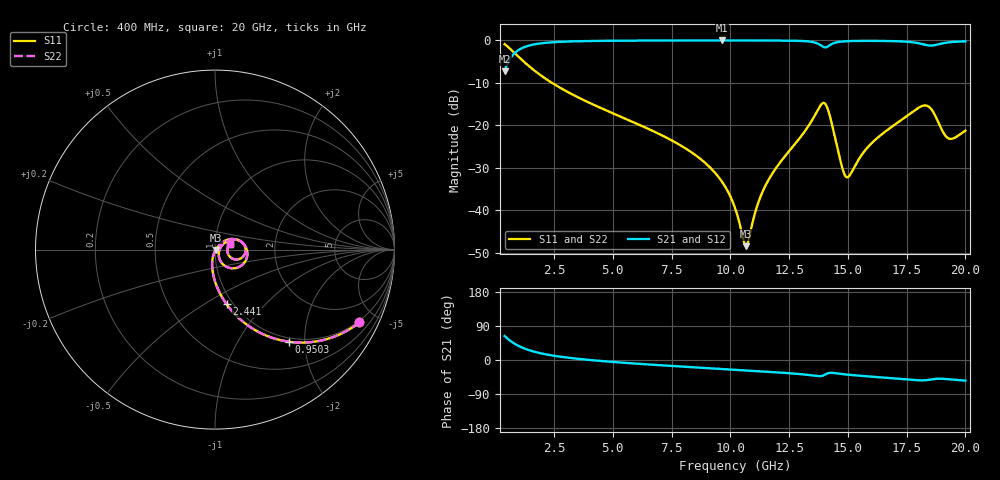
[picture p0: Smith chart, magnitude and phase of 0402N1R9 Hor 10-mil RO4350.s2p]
# GHz S MA R 50
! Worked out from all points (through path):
!   1960 points, 400 MHz to 20 GHz, reference 50 ohm
!   highest |S21| = -0.03 dB at 9.635 GHz (marker M1); lowest = -7.3 dB at 400 MHz (marker M2)
!   group delay of S21, straight-line fit = 11.7 ps
!   lowest |S11| = -48.5 dB at 10.67 GHz (marker M3), VSWR 1.01, Z = 50.3 - j0.195 ohm
!   |S11| at or under -10 dB: 2.407 GHz to end of sweep
!   |S22| runs from -48.5 to -0.9 dB; largest |S21 - S12| = 0
!   S11 on the Smith chart (normalised r, x): 400 MHz: 0.93, -4.01; 950.3 MHz: 0.93, -1.68; 2.441 GHz: 0.93, -0.63; 20 GHz: 1.18, +0.07
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0.4  0.9011 -26.7  0.4334 63.3  0.4334 63.3  0.9011 -26.7
0.9502808  0.6566 -51.4  0.7535 38.6  0.7535 38.6  0.6566 -51.4
1.560592  0.4649 -66.3  0.8843 23.6  0.8843 23.6  0.4649 -66.3
2.441041  0.312 -78.0  0.9486 11.8  0.9486 11.8  0.312 -78.0
3.671669  0.2033 -87.4  0.9773 2.1  0.9773 2.1  0.2033 -87.4
6.943338  0.07954 -101.7  0.9941 -13.5  0.9941 -13.5  0.07954 -101.7
8.594181  0.04284 -106.0  0.9959 -19.8  0.9959 -19.8  0.04284 -106.0
9.634712  0.02182 -105.2  0.9962 -23.7  0.9962 -23.7  0.02182 -105.2
10.205  0.01052 -96.5  0.9961 -25.8  0.9961 -25.8  0.01052 -96.5
10.66524  0.003756 -31.0  0.9958 -27.5  0.9958 -27.5  0.003756 -31.0
11.1755  0.01191 40.0  0.9953 -29.4  0.9953 -29.4  0.01191 40.0
11.55569  0.02087 46.1  0.9946 -30.9  0.9946 -30.9  0.02087 46.1
13.46667  0.113 31.6  0.959 -40.6  0.959 -40.6  0.113 31.6
13.86687  0.1753 1.7  0.866 -42.4  0.866 -42.4  0.1753 1.7
14.06697  0.174 -29.4  0.8267 -37.2  0.8267 -37.2  0.174 -29.4
14.76733  0.03109 -47.9  0.9688 -37.2  0.9688 -37.2  0.03109 -47.9
14.96743  0.02433 -15.9  0.9769 -38.5  0.9769 -38.5  0.02433 -15.9
15.81787  0.05382 33.4  0.9853 -43.0  0.9853 -43.0  0.05382 33.4
16.73834  0.09021 33.4  0.9808 -47.3  0.9808 -47.3  0.09021 33.4
18.28913  0.171 -1.3  0.8854 -53.6  0.8854 -53.6  0.171 -1.3
19.25962  0.07047 -10.3  0.9445 -50.6  0.9445 -50.6  0.07047 -10.3
20  0.08633 19.5  0.9719 -54.5  0.9719 -54.5  0.08633 19.5
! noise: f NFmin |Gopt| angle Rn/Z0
0.4  0.001275  0.7989  4.25  0.001312
2.571  0.005071  0.6797  8.077  0.003046
4.752  0.008078  0.6383  13.29  0.004159
6.933  0.01084  0.6151  18.58  0.00511
9.104  0.01371  0.6064  23.79  0.006184
11.29  0.0181  0.6298  28.93  0.008632
13.47  0.05531  0.8393  34.28  0.06658
15.64  0.03646  0.737  39.47  0.02463
17.82  0.07264  0.8433  44.59  0.08435
20  0.05431  0.7776  49.54  0.04134
